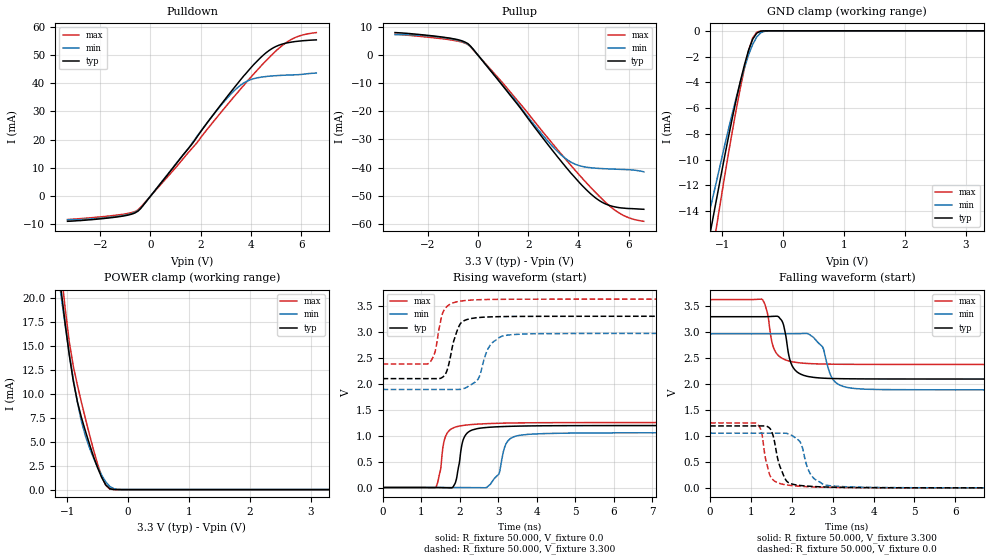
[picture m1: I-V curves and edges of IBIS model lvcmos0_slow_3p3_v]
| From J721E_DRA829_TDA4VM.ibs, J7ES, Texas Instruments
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|   slow_3p3_v
[Model]   lvcmos0_slow_3p3_v
Model_type I/O
Polarity   Non-Inverting
Enable   Active-High
Vinl = 0
Vinh = 0.8
Vmeas = 1.65
Vref = 3.3
Cref = 2pF
Rref = 100000
|   typ   min   max
C_comp   1.415pF   1.382pF   1.448pF
[Voltage Range]   3.3   2.97   3.63
[Temperature Range]   27   150   -40
[Pullup Reference]   3.3   2.97   3.63
[Pulldown Reference]   0   0   0
[Power Clamp Reference]   3.3   2.97   3.63
[GND Clamp Reference]   0   0   0
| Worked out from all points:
|   slope of the pulldown table from 0 to 0.495 V, typ, clamps not added: 89.6 ohm
|   slope of the pullup table from 0 to 0.495 V, typ, clamps not added: 90.9 ohm
|   GND clamp passes 1 mA (typ) near -0.53 V on its own axis
|   POWER clamp passes 1 mA (typ) near -0.41 V on its own axis
|   rising waveform, R_fixture 50.000, V_fixture 0.0: 20-80 % time 176ps typ, 256ps min, 171ps max; typ from 0 V to 1.19 V
|   rising waveform, R_fixture 50.000, V_fixture 3.300: 20-80 % time 250ps typ, 314ps min, 202ps max; typ from 2.1 V to 3.3 V
|   falling waveform, R_fixture 50.000, V_fixture 3.300: 20-80 % time 199ps typ, 289ps min, 196ps max; typ from 3.3 V to 2.1 V
|   falling waveform, R_fixture 50.000, V_fixture 0.0: 20-80 % time 240ps typ, 278ps min, 182ps max; typ from 1.19 V to 0 V
[Pulldown]
|Voltage   I(typ)   I(min)   I(max)
-3.3V     -8.88mA    -8.385mA   -8.25mA
-1.3V     -7.308mA   -7.119mA   -6.652mA
-500mV    -5.306mA   -5.103mA   -4.87mA
-300mV    -3.354mA   -3.386mA   -3.022mA
1.6V      17.84mA    18.03mA    16.39mA
2.7V      31.18mA    31mA       28.5mA
3.2V      36.91mA    36.13mA    33.86mA
3.6V      41.35mA    39.38mA    38.06mA
4.1V      46.49mA    41.56mA    43.15mA
4.9V      52.56mA    42.59mA    50.61mA
5.7V      54.65mA    42.94mA    55.9mA
6.6V      55.31mA    43.57mA    57.9mA
[Pullup]
|Voltage   I(typ)   I(min)   I(max)
-3.3V     8.025mA    7.28mA     7.462mA
-1.4V     6.408mA    6.261mA    5.826mA
-800mV    5.499mA    5.284mA    4.983mA
-400mV    4.1mA      3.839mA    3.763mA
1V        -11.05mA   -10.89mA   -10.06mA
2.7V      -30.85mA   -29.76mA   -28.57mA
3.5V      -39.82mA   -36.87mA   -37.14mA
4.1V      -45.93mA   -39.47mA   -43.29mA
4.6V      -50.21mA   -40.15mA   -48.11mA
5V        -52.61mA   -40.39mA   -51.69mA
5.8V      -54.41mA   -40.68mA   -57.07mA
6.6V      -54.82mA   -41.52mA   -59.1mA
[GND_clamp]
|Voltage   I(typ)   I(min)   I(max)
-3.3V     -91.93mA   -62.08mA   -135.9mA
-1.3V     -18.16mA   -15.85mA   -21.32mA
-1.233V   -16.57mA   -14.51mA   -19.39mA
-1.167V   -14.92mA   -13.18mA   -17.39mA
-1.1V     -13.23mA   -11.81mA   -15.39mA
-1.033V   -11.55mA   -10.42mA   -13.42mA
-833mV    -6.742mA   -6.382mA   -7.775mA
-633mV    -2.616mA   -2.841mA   -2.866mA
-500mV    -654.2uA   -1.063mA   -567uA
-433mV    -179.7uA   -474.3uA   -107.3uA
-233mV    -333.4nA   -7.881uA   -216.8nA
3.3V      0A         0A         0A
[POWER_clamp]
|Voltage   I(typ)   I(min)   I(max)
-3.3V     163.7mA    143.3mA    185.7mA
-1.1V     20.75mA    20.13mA    22.76mA
-1.033V   17.24mA    17.07mA    18.82mA
-967mV    14.03mA    14.18mA    15.4mA
-900mV    11.29mA    11.5mA     12.85mA
-767mV    7.523mA    7.108mA    9.097mA
-633mV    4.708mA    4.343mA    5.698mA
-500mV    2.263mA    2.325mA    2.644mA
-367mV    497.9uA    807.2uA    443.4uA
-300mV    94.26uA    333.7uA    53.33uA
-100mV    158.3nA    4.238uA    99.13nA
3.3V      0A         0A         0A
[Ramp]
| variable   typ   min   max
dV/dt_r   0.716/0.176n   0.633/0.257n   0.751/0.171n
dV/dt_f   0.721/0.199n   0.649/0.289n   0.750/0.196n
R_load = 50.000
[Rising Waveform]
R_fixture= 50.000
V_fixture= 0.0
V_fixture_min= 0.0
V_fixture_max= 0.0
|time   V(typ)   V(min)   V(max)
0s        2.233uV    22.67uV    3.142uV
1.378ns   -170.2uV   37.08uV    3.025mV
1.631ns   -3.81mV    -75.25uV   979.4mV
1.882ns   80.33mV    -80.37uV   1.163V
2.041ns   754.8mV    -747.2uV   1.19V
2.793ns   1.162V     60.76mV    1.233V
3.022ns   1.171V     269.9mV    1.238V
3.22ns    1.177V     864.7mV    1.241V
3.55ns    1.183V     1.006V     1.245V
10ns      1.194V     1.055V     1.252V
[Rising Waveform]
R_fixture= 50.000
V_fixture= 3.300
V_fixture_min= 2.970
V_fixture_max= 3.630
|time   V(typ)   V(min)   V(max)
0s        2.098V     1.889V     2.38V
1.205ns   2.098V     1.889V     2.398V
1.359ns   2.098V     1.889V     2.608V
1.55ns    2.122V     1.889V     3.344V
1.67ns    2.252V     1.889V     3.489V
1.998ns   3.132V     1.89V      3.588V
2.46ns    3.273V     2.071V     3.618V
2.769ns   3.287V     2.716V     3.624V
3.189ns   3.294V     2.931V     3.627V
10ns      3.3V       2.97V      3.63V
[Falling Waveform]
R_fixture= 50.000
V_fixture= 3.300
V_fixture_min= 2.970
V_fixture_max= 3.630
|time   V(typ)   V(min)   V(max)
0s        3.3V       2.97V      3.63V
1.279ns   3.3V       2.97V      3.632V
1.537ns   3.307V     2.97V      2.738V
1.673ns   3.3V       2.97V      2.551V
2.064ns   2.285V     2.972V     2.424V
2.528ns   2.131V     2.903V     2.393V
2.766ns   2.115V     2.696V     2.388V
3.014ns   2.108V     2.084V     2.384V
3.438ns   2.103V     1.925V     2.382V
10ns      2.098V     1.889V     2.38V
[Falling Waveform]
R_fixture= 50.000
V_fixture= 0.0
V_fixture_min= 0.0
V_fixture_max= 0.0
|time   V(typ)   V(min)   V(max)
0s        1.194V     1.055V     1.252V
1.168ns   1.194V     1.055V     1.218V
1.258ns   1.194V     1.055V     1.084V
1.443ns   1.162V     1.055V     287.1mV
1.861ns   142.9mV    1.053V     57.75mV
2.211ns   45.76mV    875.8mV    29.85mV
2.383ns   33.66mV    392.4mV    22.37mV
2.518ns   26.84mV    200mV      18.07mV
2.845ns   16.06mV    50.78mV    11.19mV
10ns      71.42uV    151.9uV    48.03uV
